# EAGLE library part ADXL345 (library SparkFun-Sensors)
Analog Devices ADXL345 3-Axis SPI/I2C 2/4/8/16g Accelerometer The ADXL345 is a small, thin, low power, 3-axis accelerometer with high resolution (13-bit) measurement at up to ±16g. Digital output data is formatted as 16-bit twos complement and is accessible through either a SPI (3- or 4-wire) or I2C digital interface. Datasheet SparkFun Products SparkFun Triple Axis Accelerometer Breakout - ADXL345 (SEN-09836) Triple Axis Accelerometer - ADXL345 (SEN-09045) SparkFun 6 Degrees of Freedom IMU Digital Combo Board - ITG3200/ADXL345 (SEN-10121)
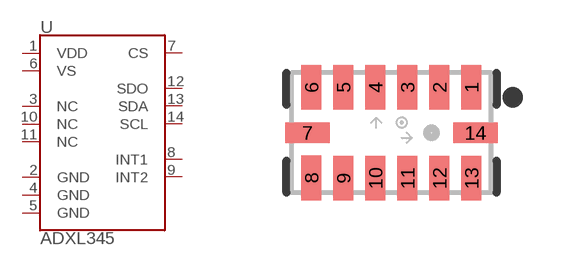
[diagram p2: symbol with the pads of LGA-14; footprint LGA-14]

Designator prefix U

## ADXL345 (PROD_ID: IC-09097; SF_ID: SEN-09045)  [LGA-14]
1  VDD
2  GND
3  NC
4  GND
5  GND
6  VS
7  CS
8  INT1
9  INT2
10  NC
11  NC
12  SDO
13  SDA
14  SCL

## Footprint LGA-14 (pad centres in mm)
14-Pin LGA (3 x 5 x 1 mm) (1:1 footprint) Datasheet Specifications: Pin Count: 14 Area: 3.0 x 5.0 x 1.0 mm Pitch: 0.8 mm Devices Using: ADXL345
smd 0.5 x 1.124: 1 2,1.138; 2 1.2,1.138; 3 0.4,1.138; 4 -0.4,1.138; 5 -1.2,1.138; 6 -2,1.138; 8 -2,-1.13; 9 -1.2,-1.138; 10 -0.4,-1.138; 11 0.4,-1.138; 12 1.2,-1.138; 13 2,-1.138
smd 1.124 x 0.5: 7 -2.1,0; 14 2.1,0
